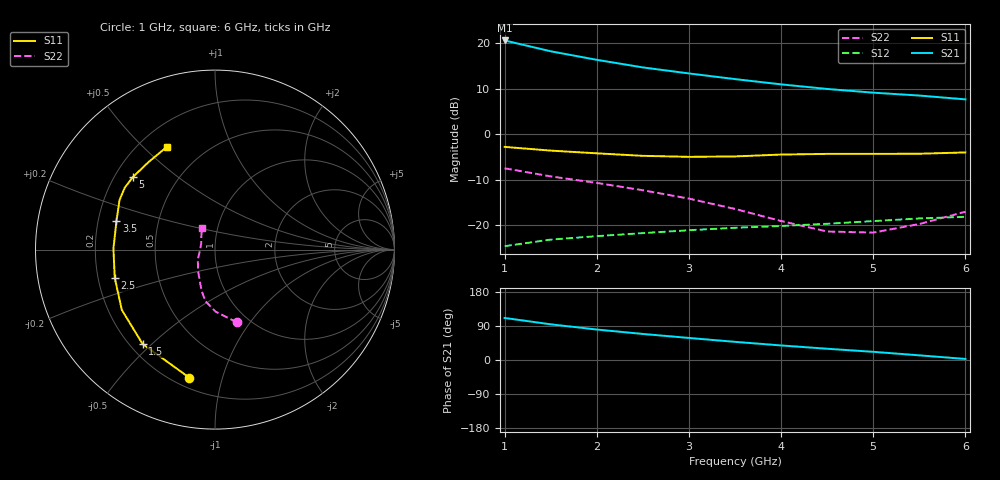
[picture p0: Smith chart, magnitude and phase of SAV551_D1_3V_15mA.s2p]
! Created Mon Oct 27 14:23:49 2008
# hz S ma R 50
! 2 Port Network Data from SP1.SP block
! freq  magS11  angS11  magS21  angS21  magS12  angS12  magS22  angS22
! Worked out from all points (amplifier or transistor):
!   11 points, 1 GHz to 6 GHz, reference 50 ohm
!   highest |S21| = 20.7 dB at 1 GHz (marker M1)
!   |S21| within 3 dB of that: start of sweep to 1.664 GHz
!   unconditionally stable (mu >= 1): 3.688 GHz to end of sweep
!   at 1.5 GHz: K = 0.50, MSG = 20.7 dB, |S12| = -23.2 dB
!   at 3.5 GHz: K = 0.98, MSG = 16.4 dB, |S12| = -20.6 dB
!   at 6 GHz: K = 1.18, MAG = 10.4 dB, |S12| = -18.1 dB
!   S11 on the Smith chart (normalised r, x): 1 GHz: 0.26, -0.79; 1.5 GHz: 0.25, -0.47; 2.5 GHz: 0.27, -0.13; 3.5 GHz: 0.28, +0.13; 5 GHz: 0.27, +0.35; 6 GHz: 0.31, +0.59
1e9  0.7281 -101.3  10.8 111.0  0.05885 38.7  0.4236 -73.2
1.5e9  0.6626 -127.5  8.209 94.1  0.06951 30.4  0.3449 -89.6
2e9  0.6184 -147.1  6.612 80.4  0.07587 24.6  0.2922 -100.4
2.5e9  0.5804 -164.2  5.453 68.7  0.08193 20.7  0.2428 -107.8
3e9  0.5659 179.5  4.683 58.2  0.08814 17.3  0.1964 -115.5
3.5e9  0.5718 163.7  4.056 47.9  0.09376 13.4  0.1512 -128.5
4e9  0.5995 152.5  3.55 38.4  0.09814 10.0  0.1113 -149.3
4.5e9  0.6099 145.4  3.16 29.7  0.1038 7.3  0.08533 -174.7
5e9  0.6105 138.6  2.876 21.6  0.1111 4.2  0.08297 158.8
5.5e9  0.6121 127.4  2.674 12.3  0.1188 -0.2  0.1032 137.7
6e9  0.6328 114.9  2.427 2.8  0.1238 -4.8  0.1409 121.3
